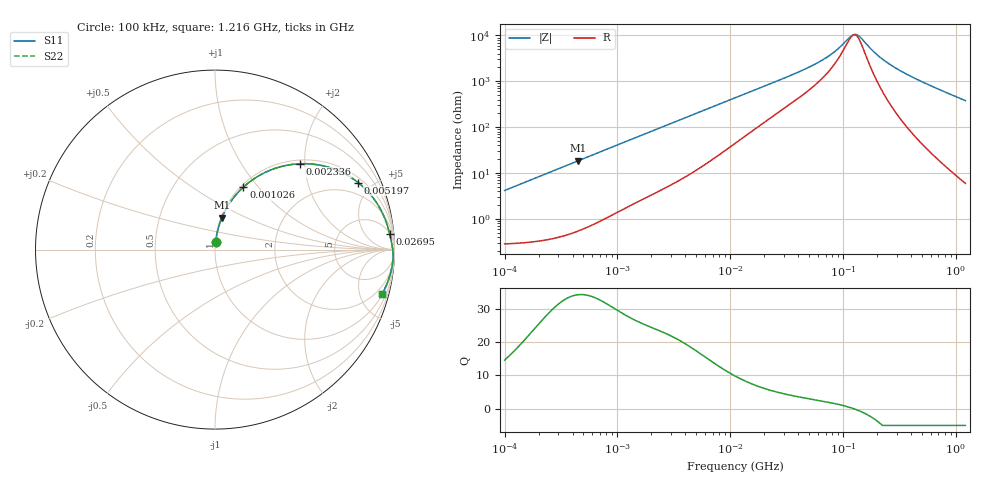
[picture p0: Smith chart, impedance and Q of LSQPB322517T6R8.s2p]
! LSQPB322517T6R8  S-PARAMETER MODEL  ( General Type )
! Model Generated by TAIYO YUDEN Corporation (http://www.ty-top.com)
! Version 2.0
! TAIYO YUDEN Control No. 100810NG22EB-FKC
! Copyright(c) 2009 TAIYO YUDEN CO.,LTD. All Rights Reserved.
! Product Description (link to TY-COMPAS)
! https://ds.yuden.co.jp/TYCOMPAS/or/detail?pn=LSQPB322517T6R8M&u=M
! Products Name : Inductors
! Characteristics :
!  Inductance : 6.8 uH , SRF(min) : 90 MHz , DC Resistance(max) : 0.324 Ohm
!  Rated Current : Saturation :1050 mA , Temp Rise : 770 mA (40 degC)
!  Case Size : 3.2 x 2.5 / 0.126 x 0.098 [mm/inch] , Thickness : 1.7 / 0.068 [mm/inch]
!  (Conditions: Temperature = 25 degC , DC Bias Current/Voltage = 0A / 0V)
! External Node Assignments :
!  1  o---GGG---o  2
! GND o---------o GND
! Frequency Range : 0.1MHz  -  1216.35853MHz  [ 402 STEP ]
# MHz S RI R 50
! Freq[MHz].  S11 Real  S11 Imag  S21 Real  S21 Imag  S12 Real  S12 Imag  S22 Real  S22 Imag
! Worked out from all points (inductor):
!   401 points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, 100 kHz to 1.216 GHz, reference 50 ohm
!   read as one part in series: L = 6.6 uH near 104.8 kHz
!   highest Q = 34.2 at 450.4 kHz (marker M1), where L = 6.58 uH
!   self-resonance near 124.3 MHz
!   S11 on the Smith chart (normalised r, x): 100 kHz: 1.01, +0.08; 1.026 MHz: 1.03, +0.84; 2.336 MHz: 1.08, +1.88; 5.197 MHz: 1.24, +4.14; 26.95 MHz: 5, +21; 1.216 GHz: 1.12, -7.57
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0.1  0.00454 0.0412  0.9955 -0.0412  0.9955 -0.0412  0.00454 0.0412
0.227742  0.0122 0.0929  0.9878 -0.0929  0.9878 -0.0929  0.0122 0.0929
0.450412  0.0384 0.1781  0.9616 -0.1781  0.9616 -0.1781  0.0384 0.1781
0.483335  0.0435 0.1899  0.9565 -0.1899  0.9565 -0.1899  0.0435 0.1899
1.025777  0.1585 0.3485  0.8415 -0.3485  0.8415 -0.3485  0.1585 0.3485
1.49436  0.2774 0.4291  0.7226 -0.4291  0.7226 -0.4291  0.2774 0.4291
2.336123  0.4713 0.4783  0.5287 -0.4783  0.5287 -0.4783  0.4713 0.4783
3.324187  0.6337 0.4586  0.3663 -0.4586  0.3663 -0.4586  0.6337 0.4586
5.196679  0.7974 0.3735  0.2026 -0.3735  0.2026 -0.3735  0.7974 0.3735
7.394617  0.879 0.291  0.121 -0.291  0.121 -0.291  0.879 0.291
11.02886  0.931 0.2077  0.069 -0.2077  0.069 -0.2077  0.931 0.2077
26.95328  0.9729 0.0891  0.0271 -0.0891  0.0271 -0.0891  0.9729 0.0891
53.30631  0.9832 0.0416  0.0168 -0.0416  0.0168 -0.0416  0.9832 0.0416
77.65708  0.9869 0.0225  0.0131 -0.0225  0.0131 -0.0225  0.9869 0.0225
91.55239  0.9882 0.0147  0.0118 -0.0147  0.0118 -0.0147  0.9882 0.0147
115.8234  0.99 0.00365  0.01 -0.00365  0.01 -0.00365  0.99 0.00365
127.2468  0.9906 -0.00088  0.00941 0.00088  0.00941 0.00088  0.9906 -0.00088
139.7969  0.9911 -0.00553  0.00886 0.00553  0.00886 0.00553  0.9911 -0.00553
194.3008  0.9924 -0.0233  0.0076 0.0233  0.0076 0.0233  0.9924 -0.0233
257.6478  0.9924 -0.0412  0.00761 0.0412  0.00761 0.0412  0.9924 -0.0412
486.1475  0.986 -0.0968  0.014 0.0968  0.014 0.0968  0.986 -0.0968
1216.359  0.9314 -0.245  0.0686 0.245  0.0686 0.245  0.9314 -0.245
